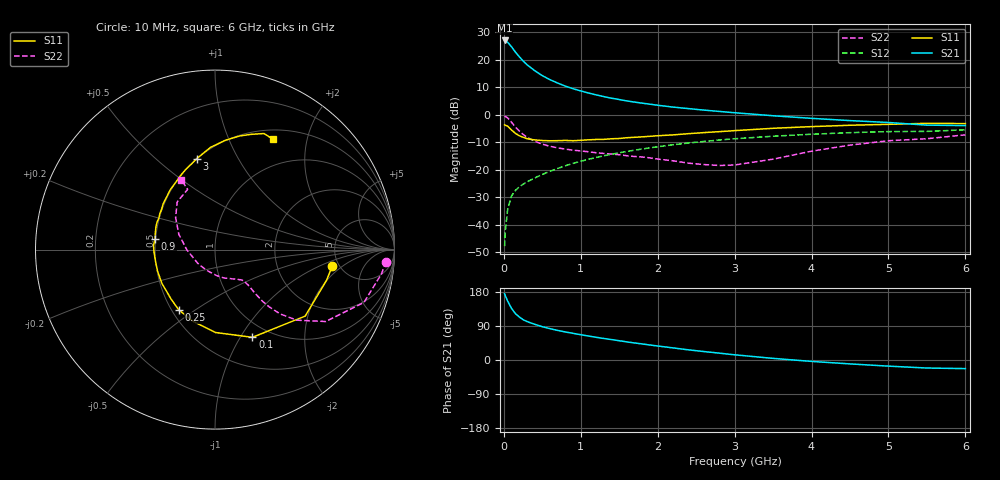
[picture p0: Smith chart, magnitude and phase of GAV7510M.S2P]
! Infineon Technologies  Discrete & RF Semiconductors
! BF775
! Si NPN RF Bipolar Junction Transistor in SOT23
! VCE = 0.75 V  IC = 10 mA
! Common Emitter S-Parameters:  May  1996
# GHz  S  MA  R  50
!  f  S11  S21  S12  S22
! GHz  MAG  ANG  MAG  ANG  MAG  ANG  MAG  ANG
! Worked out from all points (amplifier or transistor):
!   36 points, 10 MHz to 6 GHz, reference 50 ohm
!   highest |S21| = 27.1 dB at 10 MHz (marker M1)
!   |S21| within 3 dB of that: start of sweep to 118.2 MHz
!   unconditionally stable (mu >= 1): 430.2 MHz to end of sweep
!   at 250 MHz: K = 0.76, MSG = 22.4 dB, |S12| = -25.2 dB
!   at 1.4 GHz: K = 1.20, MAG = 7.5 dB, |S12| = -14.3 dB
!   at 6 GHz: K = 1.06, MAG = -0.7 dB, |S12| = -5.4 dB
!   S11 on the Smith chart (normalised r, x): 10 MHz: 4.40, -1.41; 100 MHz: 0.83, -1.13; 250 MHz: 0.54, -0.43; 900 MHz: 0.50, +0.07; 3 GHz: 0.50, +0.69; 6 GHz: 0.62, +1.47
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0.01  0.6598 -7.9  22.55 174.8  0.0041 84.5  0.9546 -4.0
0.02  0.6453 -15.1  22.28 169.4  0.0079 82.6  0.938 -8.2
0.05  0.6244 -36.4  20.88 155.1  0.0193 73.5  0.8806 -19.5
0.1  0.5312 -66.9  17.27 136.1  0.0335 62.7  0.7356 -33.0
0.15  0.462 -89.6  13.91 122.5  0.0423 57.7  0.6017 -40.8
0.2  0.418 -107.0  11.45 113.6  0.0489 56.0  0.5109 -44.6
0.25  0.3919 -120.9  9.575 106.5  0.0548 55.3  0.4418 -46.5
0.3  0.3692 -131.3  8.203 101.6  0.0602 56.2  0.3925 -47.4
0.4  0.3506 -147.5  6.387 94.3  0.0711 57.8  0.3318 -47.5
0.5  0.342 -159.1  5.169 87.9  0.0825 58.7  0.2933 -47.1
0.6  0.3379 -168.8  4.36 82.7  0.0943 59.6  0.2682 -46.9
0.7  0.3397 -177.0  3.788 78.1  0.1061 60.1  0.2513 -47.2
0.9  0.3391 170.1  2.99 70.3  0.1314 59.8  0.2284 -48.3
1.1  0.3517 159.5  2.5 63.3  0.156 58.7  0.2135 -51.6
1.3  0.3588 150.7  2.147 56.8  0.1804 57.0  0.199 -55.0
1.6  0.3843 138.9  1.792 47.8  0.2165 53.8  0.1807 -62.8
2.2  0.4326 120.7  1.385 31.9  0.2861 46.4  0.1461 -85.7
3  0.5172 101.3  1.094 13.7  0.368 35.0  0.1227 -142.3
3.5  0.5702 92.5  0.964 4.3  0.4094 27.7  0.1566 -179.3
4.5  0.6477 77.8  0.787 -10.3  0.4749 13.9  0.2823 141.0
5.5  0.7019 67.1  0.651 -21.2  0.5007 0.4  0.3687 114.4
6  0.6946 62.2  0.639 -22.7  0.5353 -3.4  0.4339 115.9
